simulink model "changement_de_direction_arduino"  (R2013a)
settings: Solver=ode45  StartTime=0.0  StopTime=inf  RelTol=1e-3
libraries: arduino_io_lib x6

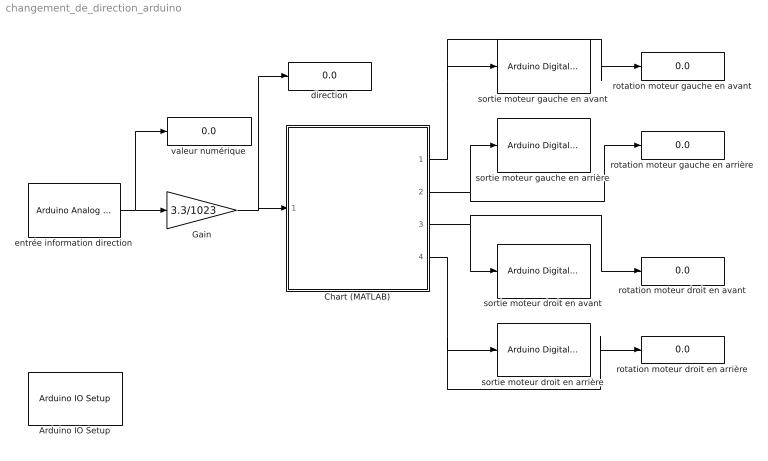
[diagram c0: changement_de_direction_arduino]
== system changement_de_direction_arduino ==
  Arduino IO Setup : arduino_io_lib/Arduino IO Setup  Priority=3  arduinoVar=Temporary arduino variable: Arduino1  workspaceVarName=a  comPort=COM4
  Chart (MATLAB) : Stateflow chart  TreatAsAtomicUnit=on
  Gain : Gain  Gain=3.3/1023
  direction : Display
  entrée information direction : arduino_io_lib/Arduino Analog Read  arduinoVar=Temporary arduino variable: Arduino1  arduinoPin=0  T=0.2
  rotation moteur droit en arrière : Display
  rotation moteur droit en avant : Display
  rotation moteur gauche en arrière : Display
  rotation moteur gauche en avant : Display
  sortie moteur droit en arrière : arduino_io_lib/Arduino Digital Write  arduinoVar=Temporary arduino variable: Arduino1  arduinoPin=2  T=0.2
  sortie moteur droit en avant : arduino_io_lib/Arduino Digital Write  arduinoVar=Temporary arduino variable: Arduino1  arduinoPin=3  T=0.2
  sortie moteur gauche en arrière : arduino_io_lib/Arduino Digital Write  arduinoVar=Temporary arduino variable: Arduino1  arduinoPin=4  T=0.2
  sortie moteur gauche en avant : arduino_io_lib/Arduino Digital Write  arduinoVar=Temporary arduino variable: Arduino1  arduinoPin=5  T=0.2
  valeur numérique : Display
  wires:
  entrée information direction/1 -> valeur numérique/1, Gain/1
  Gain/1 -> direction/1, Chart (MATLAB)/1(direction)
  Chart (MATLAB)/1(mgav) -> sortie moteur gauche en avant/1, rotation moteur gauche en avant/1
  Chart (MATLAB)/4(mdar) -> sortie moteur droit en arrière/1, rotation moteur droit en arrière/1
  Chart (MATLAB)/2(mgar) -> rotation moteur gauche en arrière/1, sortie moteur gauche en arrière/1
  Chart (MATLAB)/3(mdav) -> rotation moteur droit en avant/1, sortie moteur droit en avant/1
